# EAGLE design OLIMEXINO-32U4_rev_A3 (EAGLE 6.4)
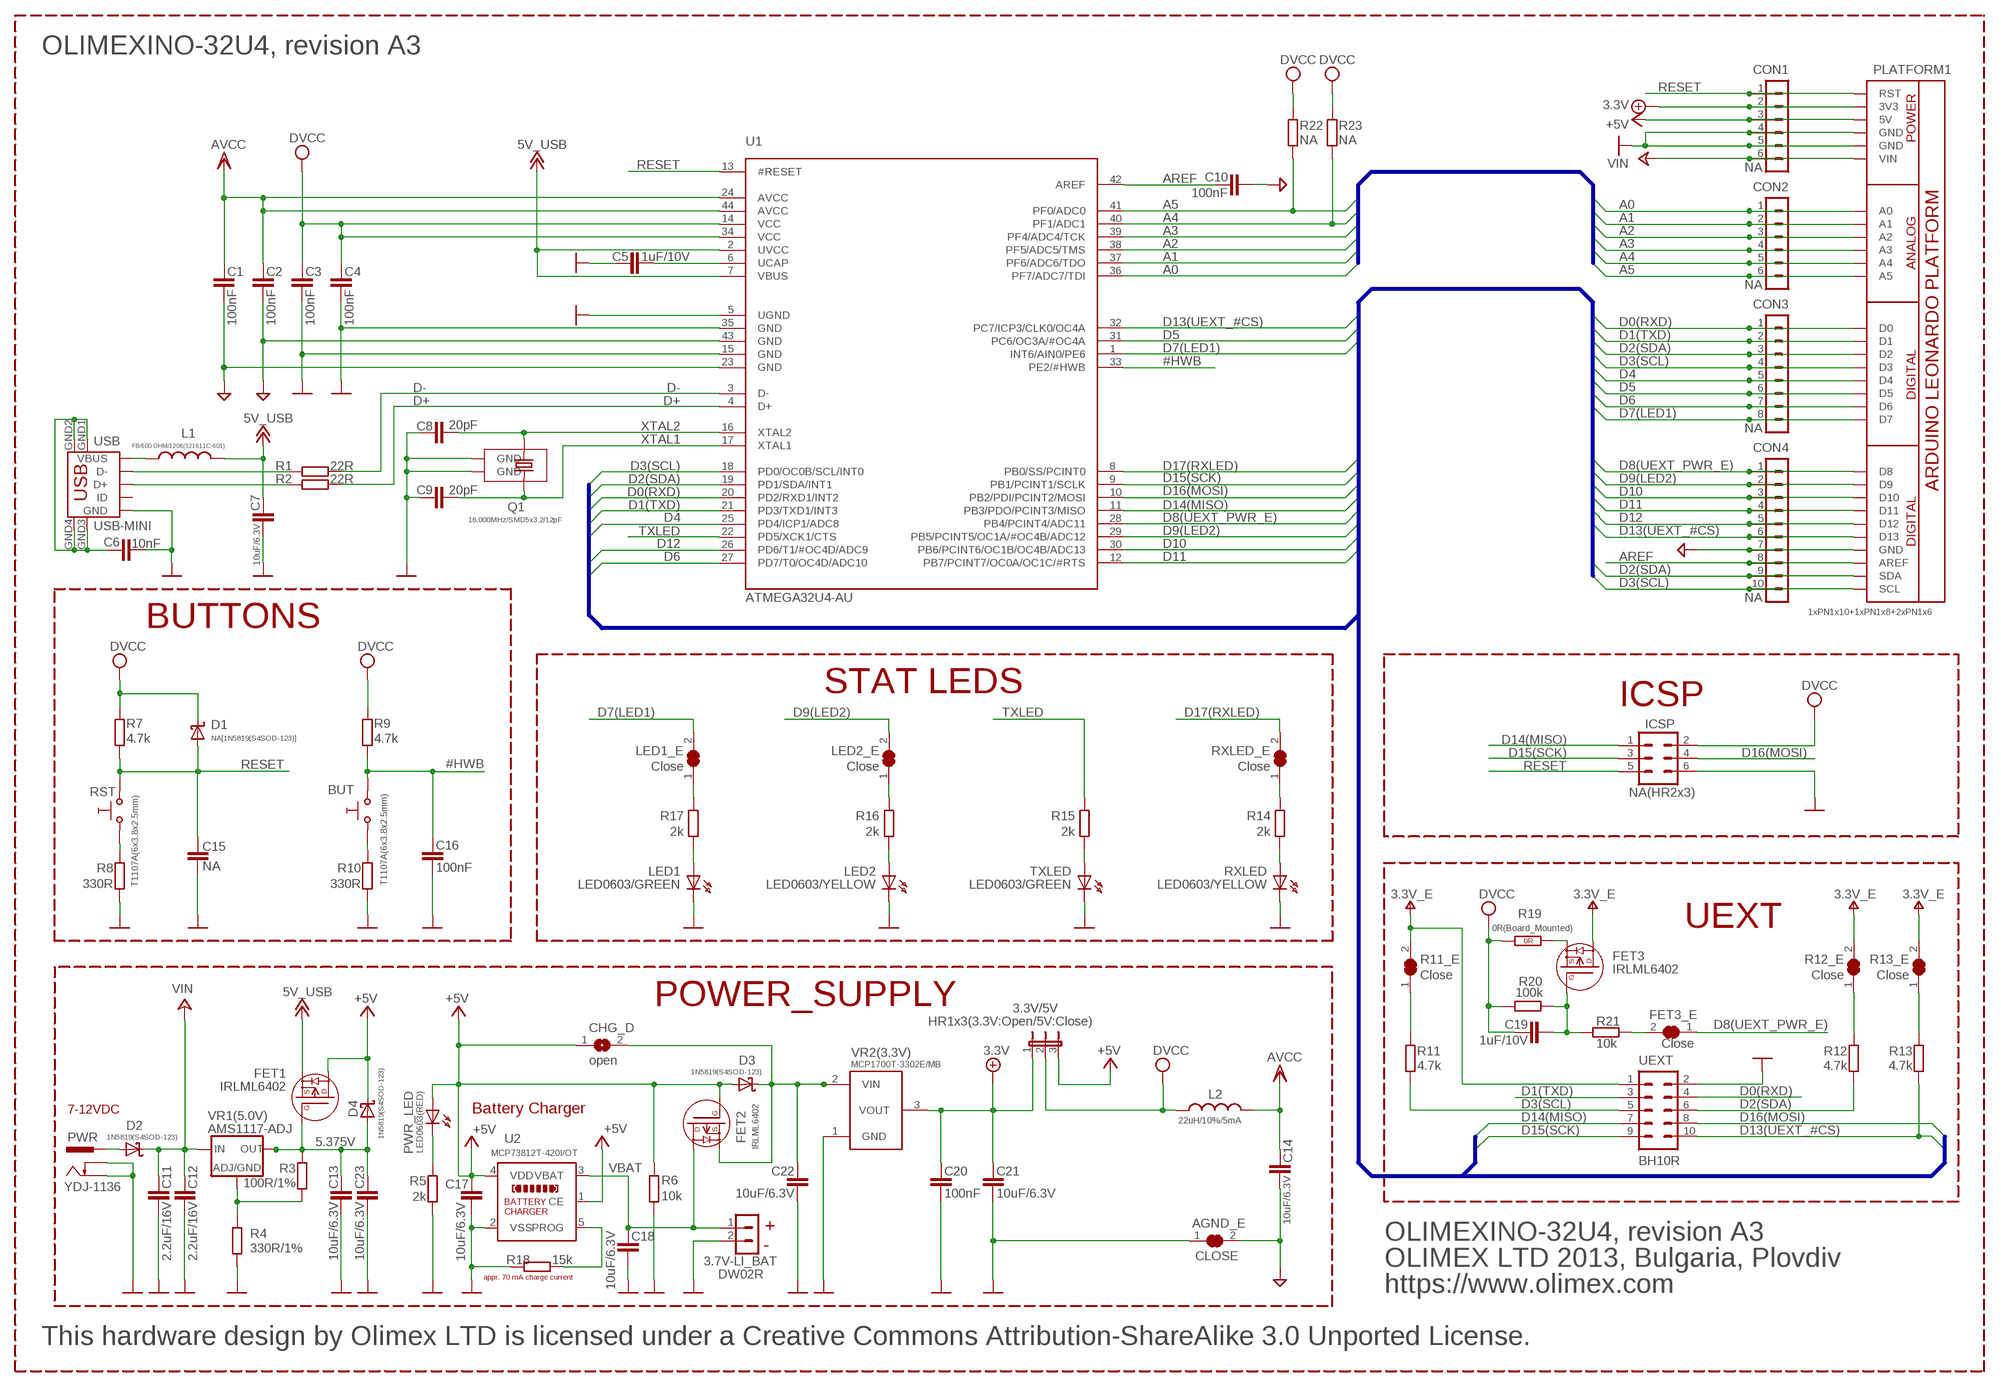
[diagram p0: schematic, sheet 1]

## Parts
3.3V/5V  HR1x3(3.3V:Open/5V:Close)  JP2EHR1X3  [HR1X3]
3.7V-LI_BAT  DW02R  CON2DW02R  [DW02R]
AGND_E  CLOSE  SJSJ_1_SMALLER_CLOSE  [SJ_1_SMALLER_CLOSE]
BUT  T1107A(6x3.8x2.5mm)  SW-TAKT6  [SW-TAKT_6X3.5_SMD]
C1  100nF  C-EUC0603_DWS  [C0603_DWS]
C2  100nF  C-EUC0603_DWS  [C0603_DWS]
C3  100nF  C-EUC0603_DWS  [C0603_DWS]
C4  100nF  C-EUC0603_DWS  [C0603_DWS]
C5  1uF/10V  C-EUC0603_DWS  [C0603_DWS]
C6  10nF  C-EUC0603_DWS  [C0603_DWS]
C7  10uF/6.3V  C-EUC0603_DWS  [C0603_DWS]
C8  20pF  C-EUC0603_DWS  [C0603_DWS]
C9  20pF  C-EUC0603_DWS  [C0603_DWS]
C10  100nF  C-EUC0603_DWS  [C0603_DWS]
C11  2.2uF/16V  C-EUC0805_5MIL_DWS  [C0805_5MIL_DWS]
C12  2.2uF/16V  C-EUC0805_5MIL_DWS  [C0805_5MIL_DWS]
C13  10uF/6.3V  C-EUC0603_DWS  [C0603_DWS]
C14  10uF/6.3V  C-EUC0603_DWS  [C0603_DWS]
C15  NA  C-EUC0603_DWS  [C0603_DWS]
C16  100nF  C-EUC0603_DWS  [C0603_DWS]
C17  10uF/6.3V  C-EUC0603_DWS  [C0603_DWS]
C18  10uF/6.3V  C-EUC0603_DWS  [C0603_DWS]
C19  1uF/10V  C-EUC0603_DWS  [C0603_DWS]
C20  100nF  C-EUC0603_DWS  [C0603_DWS]
C21  10uF/6.3V  C-EUC0603_DWS  [C0603_DWS]
C22  10uF/6.3V  C-EUC0603_DWS  [C0603_DWS]
C23  10uF/6.3V  C-EUC0603_DWS  [C0603_DWS]
CHG_D  open  SJSJ_SMALLER  [SJ_1_SMALLER]
CON1  NA  CON6HN1X6  [HN1X6]
CON2  NA  CON6HN1X6  [HN1X6]
CON3  NA  CON8HN1X8  [HN1X8]
CON4  NA  CON10HN1X10  [HN1X10]
D1  NA[1N5819(S4SOD-123)]  SCHOTKKY7.62SS-1N5819(S4SOD-123)  [SOD-123]
D2  1N5819(S4SOD-123)  SCHOTKKY7.62SS-1N5819(S4SOD-123)  [SOD-123]
D3  1N5819(S4SOD-123)  SCHOTKKY7.62SS-1N5819(S4SOD-123)  [SOD-123]
D4  1N5819(S4SOD-123)  SCHOTKKY7.62SS-1N5819(S4SOD-123)  [SOD-123]
FET1  IRLML6402  P-MOS+DIODIRLML6402  [SOT23]
FET2  IRLML6402  P-MOS+DIODIRLML6402  [SOT23]
FET3  IRLML6402  P-MOS+DIODIRLML6402  [SOT23]
FET3_E  Close  SJSJ_1_SMALLER_CLOSE  [SJ_1_SMALLER_CLOSE]
ICSP  NA(HR2x3)  ML6HN2X3R  [HN2X3R]
L1  FB/600 OHM/1206(321611C-601)  L-USL3216C  [L3216C]
L2  22uH/10%/5mA  L-USL3216C  [L3216C]
LED1  LED0603/GREEN  LED0603DWS  [LED-0603]
LED1_E  Close  SJSJ_1_SMALLER_CLOSE  [SJ_1_SMALLER_CLOSE]
LED2  LED0603/YELLOW  LED0603DWS  [LED-0603]
LED2_E  Close  SJSJ_1_SMALLER_CLOSE  [SJ_1_SMALLER_CLOSE]
PLATFORM1  1xPN1x10+1xPN1x8+2xPN1x6  ARDUINO_LEONARDO  [ARDUINO-LEONARDO-PLATFORM]
PWR  YDJ-1136  PWR-JAKPWR_JACK_UNI_MILLING  [PWR_JACK_UNI_MILLING]
PWR_LED  LED0603(RED)  LED0603DWS  [LED-0603]
Q1  16.000MHz/SMD5x3.2/12pF  SMALL_SMD_CRYSTAL  [CRYSTAL_SMD]
R1  22R  R-EU_R0603_5MIL_DWS  [R0603_5MIL_DWS]
R2  22R  R-EU_R0603_5MIL_DWS  [R0603_5MIL_DWS]
R3  100R/1%  R-EU_R0603_5MIL_DWS  [R0603_5MIL_DWS]
R4  330R/1%  R-EU_R0603_5MIL_DWS  [R0603_5MIL_DWS]
R5  2k  R-EU_R0603_5MIL_DWS  [R0603_5MIL_DWS]
R6  10k  R-EU_R0603_5MIL_DWS  [R0603_5MIL_DWS]
R7  4.7k  R-EU_R0603_5MIL_DWS  [R0603_5MIL_DWS]
R8  330R  R-EU_R0603_5MIL_DWS  [R0603_5MIL_DWS]
R9  4.7k  R-EU_R0603_5MIL_DWS  [R0603_5MIL_DWS]
R10  330R  R-EU_R0603_5MIL_DWS  [R0603_5MIL_DWS]
R11  4.7k  R-EU_R0603_5MIL_DWS  [R0603_5MIL_DWS]
R11_E  Close  SJSJ_1_SMALLER_CLOSE  [SJ_1_SMALLER_CLOSE]
R12  4.7k  R-EU_R0603_5MIL_DWS  [R0603_5MIL_DWS]
R12_E  Close  SJSJ_1_SMALLER_CLOSE  [SJ_1_SMALLER_CLOSE]
R13  4.7k  R-EU_R0603_5MIL_DWS  [R0603_5MIL_DWS]
R13_E  Close  SJSJ_1_SMALLER_CLOSE  [SJ_1_SMALLER_CLOSE]
R14  2k  R-EU_R0603_5MIL_DWS  [R0603_5MIL_DWS]
R15  2k  R-EU_R0603_5MIL_DWS  [R0603_5MIL_DWS]
R16  2k  R-EU_R0603_5MIL_DWS  [R0603_5MIL_DWS]
R17  2k  R-EU_R0603_5MIL_DWS  [R0603_5MIL_DWS]
R18  15k  R-EU_R0603_5MIL_DWS  [R0603_5MIL_DWS]
R19  0R(Board_Mounted)  R_0R0R(NA)  [0603_0R]
R20  100k  R-EU_R0603_5MIL_DWS  [R0603_5MIL_DWS]
R21  10k  R-EU_R0603_5MIL_DWS  [R0603_5MIL_DWS]
R22  NA  R-EU_R0603_5MIL_DWS  [R0603_5MIL_DWS]
R23  NA  R-EU_R0603_5MIL_DWS  [R0603_5MIL_DWS]
RST  T1107A(6x3.8x2.5mm)  SW-TAKT6  [SW-TAKT_6X3.5_SMD]
RXLED  LED0603/YELLOW  LED0603DWS  [LED-0603]
RXLED_E  Close  SJSJ_1_SMALLER_CLOSE  [SJ_1_SMALLER_CLOSE]
TXLED  LED0603/GREEN  LED0603DWS  [LED-0603]
U1  ATMEGA32U4-AU  ATMEGA32U4U  [TQFP44]
U2  MCP73812T-420I/OT  MCP7381XSOT-23-5  [SOT-23-5]
UEXT  BH10R  ML10R  [BH10R]
USB  USB-MINI  MINI_USB9  [USB_MINI_9PIN]
VR1(5.0V)  AMS1117-ADJ  LM1117  [SOT223]
VR2(3.3V)  MCP1700T-3302E/MB  MCP1700-REP1  [SOT89_REP_THERMALOFF]

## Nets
3.3V_REG_IN: C22.1 CHG_D.2 D3.C FET2.2(S) VR2(3.3V).2(VIN) VR2(3.3V).P$2(VIN1)
5.375V: C13.1 C23.1 D4.A FET1.1(G) R3.2 VR1(5.0V).2(OUT) VR1(5.0V).4(RAD)
#HWB: BUT.P$2 C16.1 R9.2 U1.33(PE2/#HWB)
+5V: 3.3V/5V.3 C17.1 CHG_D.1 CON1.3 D3.A D4.C FET1.3(D) FET2.1(G) PLATFORM1.5V PWR_LED.A R6.1 U2.1(CE) U2.4(VDD)
+5V/1: 3.3V/5V.1 C20.1 C21.1 CON1.2 PLATFORM1.3V3 VR2(3.3V).3(VOUT) ; supply symbol labelled 3.3V
+12V: C7.1 FET1.2(S) L1.2 U1.2(UVCC) U1.7(VBUS) ; supply symbol labelled 5V_USB
+24V: C11.1 C12.1 CON1.6 D2.C PLATFORM1.VIN VR1(5.0V).3(IN) ; supply symbol labelled VIN
A0: CON2.1 PLATFORM1.A0 U1.36(PF7/ADC7/TDI)
A1: CON2.2 PLATFORM1.A1 U1.37(PF6/ADC6/TDO)
A2: CON2.3 PLATFORM1.A2 U1.38(PF5/ADC5/TMS)
A3: CON2.4 PLATFORM1.A3 U1.39(PF4/ADC4/TCK)
A4: CON2.5 PLATFORM1.A4 R23.1 U1.40(PF1/ADC1)
A5: CON2.6 PLATFORM1.A5 R22.1 U1.41(PF0/ADC0)
AGND: AGND_E.2 C1.2 C2.2 C10.2 C14.2 CON4.7 PLATFORM1.GND@2(GND) U1.23(GND) U1.43(GND)
AREF: C10.1 CON4.8 PLATFORM1.AREF U1.42(AREF)
D0(RXD): CON3.1 PLATFORM1.D0 U1.20(PD2/RXD1/INT2) UEXT.4
D1(TXD): CON3.2 PLATFORM1.D1 U1.21(PD3/TXD1/INT3) UEXT.3
D2(SDA): CON3.3 CON4.9 PLATFORM1.D2 PLATFORM1.SDA R12.1 U1.19(PD1/SDA/INT1) UEXT.6
D3(SCL): CON3.4 CON4.10 PLATFORM1.D3 PLATFORM1.SCL R11.1 U1.18(PD0/OC0B/SCL/INT0) UEXT.5
D4: CON3.5 PLATFORM1.D4 U1.25(PD4/ICP1/ADC8)
D5: CON3.6 PLATFORM1.D5 U1.31(PC6/OC3A/#OC4A)
D6: CON3.7 PLATFORM1.D6 U1.27(PD7/T0/OC4D/ADC10)
D7(LED1): CON3.8 LED1_E.2 PLATFORM1.D7 U1.1(INT6/AIN0/PE6)
D8(UEXT_PWR_E): CON4.1 FET3_E.1 PLATFORM1.D8 U1.28(PB4/PCINT4/ADC11)
D9(LED2): CON4.2 LED2_E.2 PLATFORM1.D9 U1.29(PB5/PCINT5/OC1A/#OC4B/ADC12)
D10: CON4.3 PLATFORM1.D10 U1.30(PB6/PCINT6/OC1B/OC4B/ADC13)
D11: CON4.4 PLATFORM1.D11 U1.12(PB7/PCINT7/OC0A/OC1C/#RTS)
D12: CON4.5 PLATFORM1.D12 U1.26(PD6/T1/#OC4D/ADC9)
D13(UEXT_#CS): CON4.6 PLATFORM1.D13 R13.1 U1.32(PC7/ICP3/CLK0/OC4A) UEXT.10
D14(MISO): ICSP.1 U1.11(PB3/PDO/PCINT3/MISO) UEXT.7
D15(SCK): ICSP.3 U1.9(PB1/PCINT1/SCLK) UEXT.9
D16(MOSI): ICSP.4 U1.10(PB2/PDI/PCINT2/MOSI) UEXT.8
D17(RXLED): RXLED_E.2 U1.8(PB0/SS/PCINT0)
D+: R2.2 U1.4(D+)
D-: R1.2 U1.3(D-)
GND [pwr]: 3.7V-LI_BAT.2 AGND_E.1 C3.2 C4.2 C5.1 C6.2 C7.2 C8.1 C9.1 C11.2 C12.2 C13.2 C15.2 C16.2 C17.2 C18.2 C20.2 C21.2 C22.2 C23.2 CON1.4 CON1.5 ICSP.6 LED1.C LED2.C PLATFORM1.GND PLATFORM1.GND@1(GND) PWR.- PWR.-- Q1.NC_1(GND) Q1.NC_2(GND) R4.1 R5.2 R6.2 R8.1 R10.1 R18.1 RXLED.C TXLED.C U1.5(UGND) U1.15(GND) U1.35(GND) U2.2(VSS) UEXT.2 USB.GND VR2(3.3V).1(GND)
N$1: R1.1 USB.D-
N$2: R14.2 RXLED_E.1
N$3: R2.1 USB.D+
N$4: R11.2 R11_E.1
N$5: R15.1 TXLED.A
N$6: FET3_E.2 R21.2
N$8: R13.2 R13_E.1
N$9: LED1.A R17.1
N$11 [pwr]: R8.2 RST.P$2
N$12: BUT.P$1 R10.2
N$13: R12.2 R12_E.1
N$15: LED1_E.1 R17.2
N$16: D2.A PWR.+
N$17: LED2.A R16.1
N$18: LED2_E.1 R16.2
N$19: C19.2 FET3.1(G) R20.2 R21.1
N$20: FET3.2(S) R19.2(1.2)
N$21: PWR_LED.C R5.1
N$22: R18.2 U2.5(PROG)
N$23: R14.1 RXLED.A
N$118: C6.1 USB.GND1 USB.GND2 USB.GND3 USB.GND4
RESET: C15.1 CON1.1 D1.A ICSP.5 PLATFORM1.RST R7.2 RST.P$1 U1.13(#RESET)
TXLED: R15.2 U1.22(PD5/XCK1/CTS)
UCAP: C5.2 U1.6(UCAP)
V+: FET3.3(D) R11_E.2 R12_E.2 R13_E.2 UEXT.1 ; supply symbol labelled 3.3V_E
VBAT: 3.7V-LI_BAT.1 C18.1 FET2.3(D) U2.3(VBAT)
VBUS: L1.1 USB.VBUS
VCC: 3.3V/5V.2 C3.1 C4.1 C19.1 D1.C ICSP.2 L2.1 R7.1 R9.1 R19.1(1.1) R20.1 R22.2 R23.2 U1.14(VCC) U1.34(VCC) ; supply symbol labelled DVCC
VDD: C1.1 C2.1 C14.1 L2.2 U1.24(AVCC) U1.44(AVCC) ; supply symbol labelled AVCC
VR1_ADJ: R3.1 R4.2 VR1(5.0V).1(ADJ/GND)
XTAL1: C9.2 Q1.1 U1.17(XTAL1)
XTAL2: C8.2 Q1.2 U1.16(XTAL2)
Unconnected: USB.ID

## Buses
A[0..5]
D0(RXD),D1(TXD),D2(SDA),D3(SCL),D[4..6],D7(LED1),D8(UEXT_PWR_E),D9(LED2),D[10..12],D13(UEXT_#CS),D14(RXLED),D15(SCK),D16(MOSI),D17(MISO)

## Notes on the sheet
- OLIMEXINO-32U4, revision A3
- BUTTONS
- STAT LEDS
- ICSP
- UEXT
- POWER_SUPPLY
- 7-12VDC | Battery Charger
- +
- - | OLIMEXINO-32U4, revision A3
- OLIMEX LTD 2013, Bulgaria, Plovdiv
- appr. 70 mA charge current
- https://www.olimex.com
- This hardware design by Olimex LTD is licensed under a Creative Commons Attribution-ShareAlike 3.0 Unported License.

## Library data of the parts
3.3V/5V = jumper:JP2E: JUMPER
3.7V-LI_BAT = Penko:CON2
AGND_E CHG_D FET3_E LED1_E LED2_E R11_E R12_E R13_E RXLED_E = jumper:SJ: SMD solder JUMPER
BUT RST = gogo:SW-TAKT
C1-C23 = rcl:C-EU: CAPACITOR, European symbol
CON1 CON2 = Penko:CON6: CONNECTORS - 6 PINS
CON3 = Penko:CON8
CON4 = Penko:CON10
D1-D4 = gogo:SCHOTKKY7.62SS
FET1-FET3 = Penko:P-MOS+DIOD
ICSP = con-harting-ml:ML6: HARTING
L1 L2 = rcl:L-US: INDUCTOR, American symbol
LED1 LED2 PWR_LED RXLED TXLED = DOUBLE-SIDE:LED
PLATFORM1 = OLIMEX_CASES:ARDUINO_LEONARDO
PWR = gogo:PWR-JAK
Q1 = OLIMEX_DISCRET:SMALL_SMD_CRYSTAL
R1-R18 R20-R23 = rcl:R-EU_: RESISTOR, European symbol
R19 = OLIMEX_DISCRET:R_0R
U1 = OLIMEX_IC:ATMEGA32U4: 8-bit Microcontroller with 16/32K Bytes of ISP Flash and USB Controller
U2 = OLIMEX_DISCRET:MCP7381X
UEXT = con-harting-ml:ML10: HARTING
USB = OLIMEX_CONNECTORS:MINI_USB9
VR1(5.0V) = arm:LM1117
VR2(3.3V) = OLIMEX_DISCRET:MCP1700-REP

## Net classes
1 pwr: width 0.25 mm

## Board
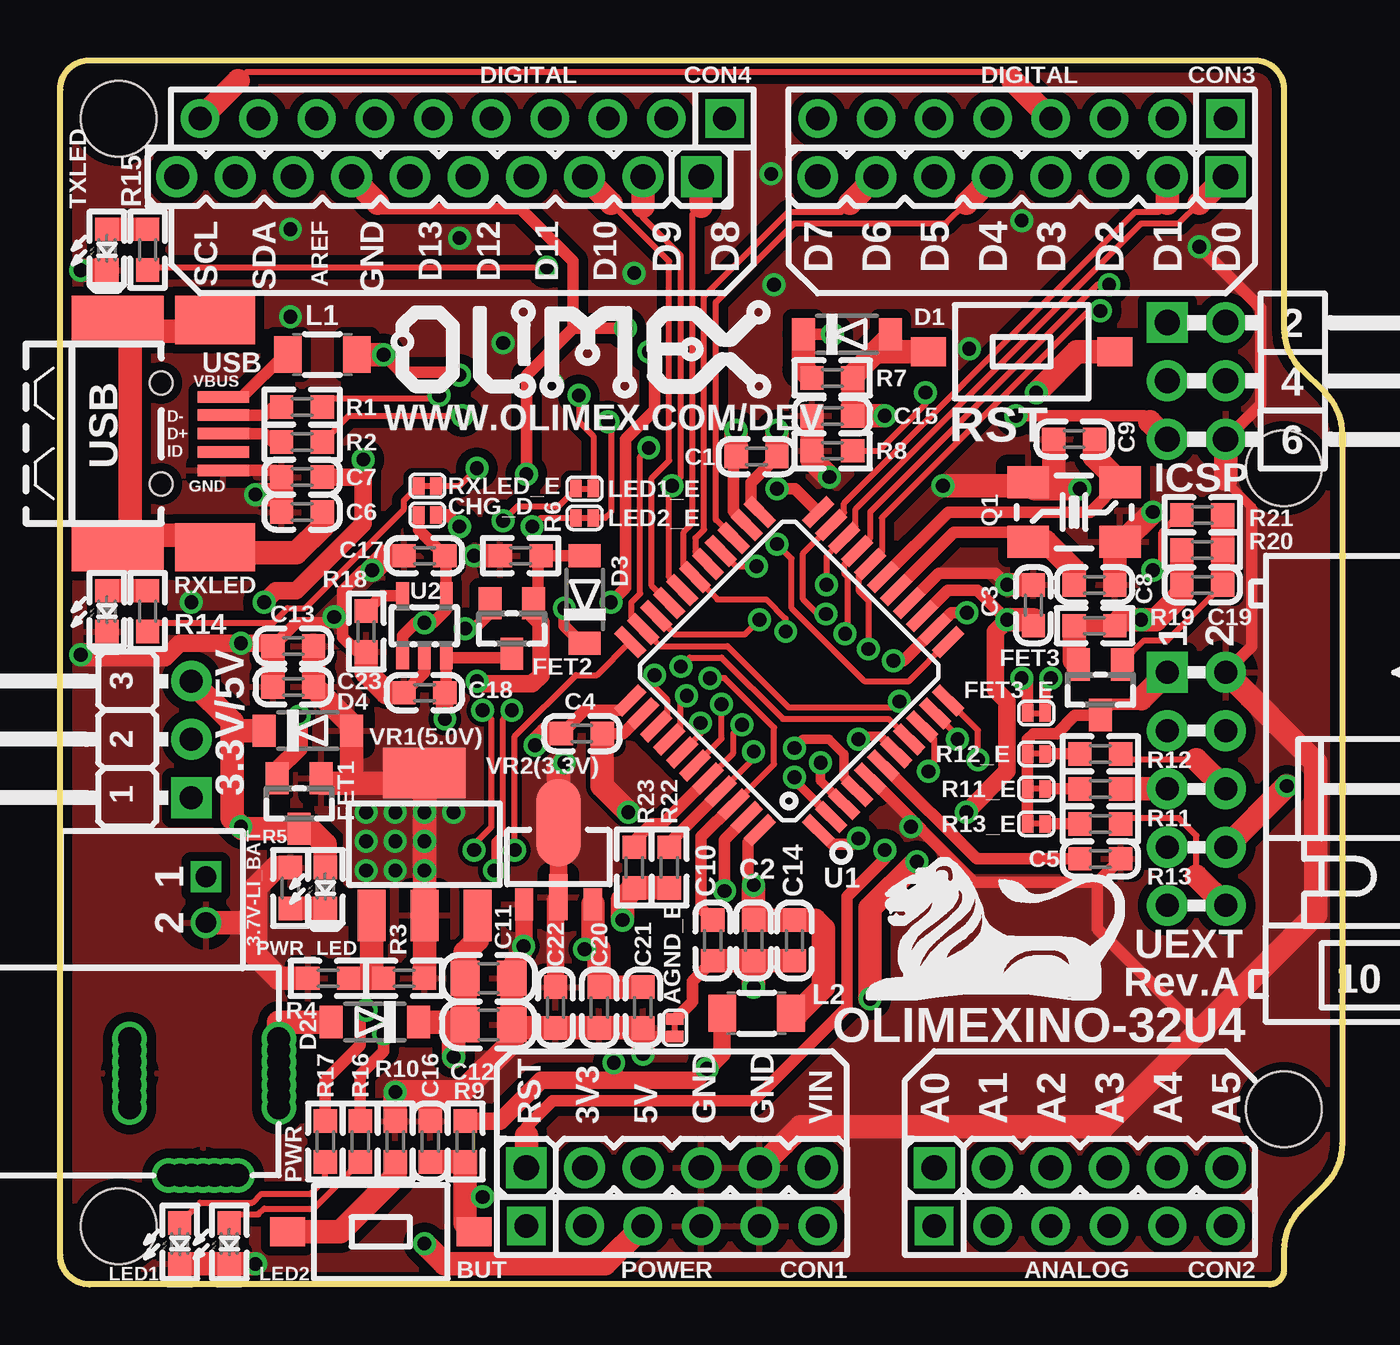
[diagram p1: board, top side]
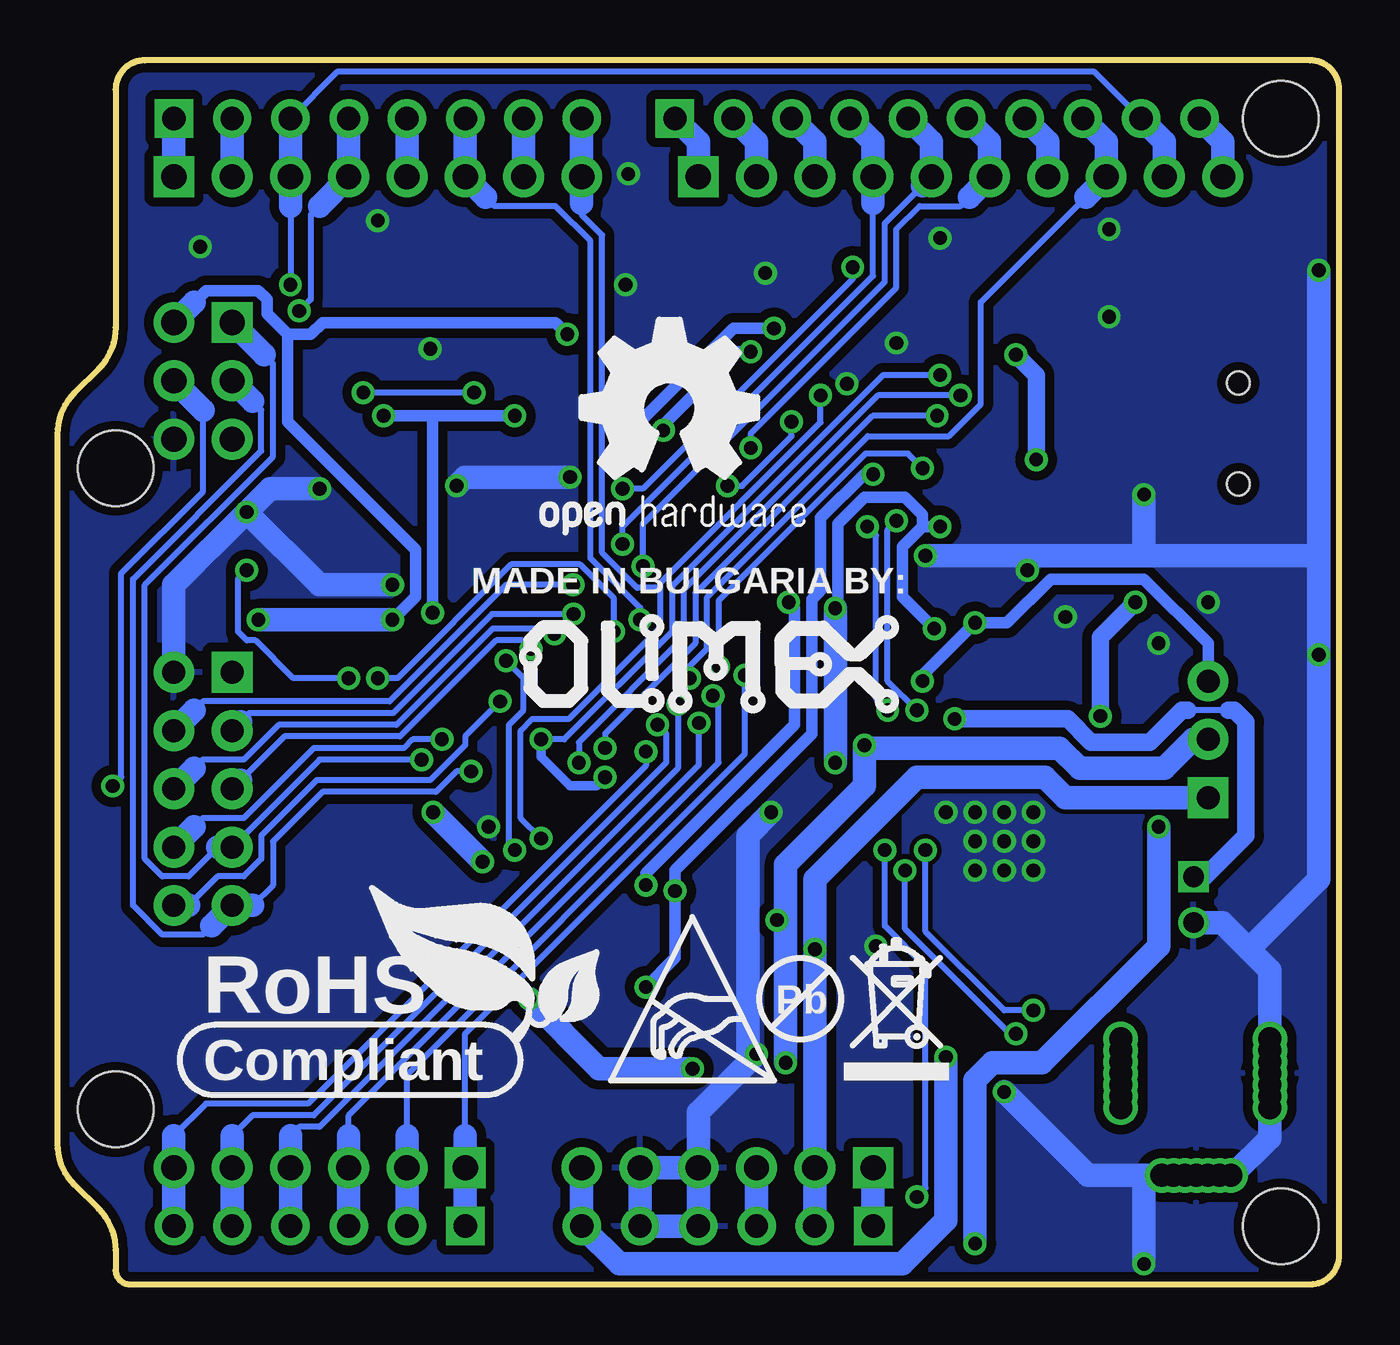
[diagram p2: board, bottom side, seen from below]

Size 55.88 x 53.34 mm. Coordinates in mm from the lower left corner, seen from the top.
Copper layers (1+16): Top 0.035mm / dielectric 1.5mm / Bottom 0.035mm
Design rules "default": minimum track width 10mil, minimum drill 0.6mm, track to track 0.2mm, track to pad 0.2mm, pad to pad 0.2mm, via to via 0.2mm, smd to smd 1mil, copper to edge 10mil, drill to drill 8mil, minimum pad ring 8mil, minimum via ring 0.2mm, stop-mask expansion 4mil, vias tented up to drill 25mil, thermal gap 20mil

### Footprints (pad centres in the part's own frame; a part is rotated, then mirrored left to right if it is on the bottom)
HR1X3 = drill 1 pad 1.778 square: 1 -2.54,0 | drill 1 pad 1.778: 2 0,0; 3 2.54,0
DW02R = drill 0.9 square: 1 -1,0 | drill 0.9: 2 1,0
SJ_1_SMALLER_CLOSE = smd 0.508 x 0.762: 1 -0.381,0; 2 0.381,0
SW-TAKT_6X3.5_SMD = smd 1.27 x 1.524: P$1 0,4.064; P$2 0,-4.064
C0603_DWS = smd 1.016 x 1.016: 1 -0.889,0; 2 0.889,0
C0805_5MIL_DWS = smd 1.27 x 1.524: 1 -1.016,0; 2 1.016,0
SJ_1_SMALLER = smd 0.508 x 0.762: 1 -0.381,0; 2 0.381,0
HN1X6 = drill 1.1 pad 1.778 square: 1 -6.35,0 | drill 1.1 pad 1.778: 2 -3.81,0; 3 -1.27,0; 4 1.27,0; 5 3.81,0; 6 6.35,0
HN1X8 = drill 1.1 pad 1.778 square: 1 -8.89,0 | drill 1.1 pad 1.778: 2 -6.35,0; 3 -3.81,0; 4 -1.27,0; 5 1.27,0; 6 3.81,0; 7 6.35,0; 8 8.89,0
HN1X10 = drill 1.1 pad 1.778 square: 1 -11.43,0 | drill 1.1 pad 1.778: 2 -8.89,0; 3 -6.35,0; 4 -3.81,0; 5 -1.27,0; 6 1.27,0; 7 3.81,0; 8 6.35,0; 9 8.89,0; 10 11.43,0
SOD-123 = smd 1 x 1.4: A 1.9,0; C -1.9,0
SOT23 = smd 1 x 1.4: 1 -0.95,-1.1; 2 0.95,-1.1; 3 0,1.1
HN2X3R = drill 1.1 pad 1.778 square: 1 -2.54,-1.27 | drill 1.1 pad 1.778: 2 -2.54,1.27; 3 0,-1.27; 4 0,1.27; 5 2.54,-1.27; 6 2.54,1.27
L3216C = smd 1.2 x 1.6: 1 -1.5,0; 2 1.5,0
LED-0603 = smd 1.016 x 1.016: A 0.889,0; C -0.889,0
ARDUINO-LEONARDO-PLATFORM = drill 1.016 pad 1.676: 3V3 22.86,2.54; 5V 25.4,2.54; A1 40.64,2.54; A2 43.18,2.54; A3 45.72,2.54; A4 48.26,2.54; A5 50.8,2.54; AREF 11.176,50.8; D1 48.26,50.8; D2 45.72,50.8; D3 43.18,50.8; D4 40.64,50.8; D5 38.1,50.8; D6 35.56,50.8; D7 33.02,50.8; D9 26.416,50.8; D10 23.876,50.8; D11 21.336,50.8; D12 18.796,50.8; D13 16.256,50.8; GND 27.94,2.54; GND@1 30.48,2.54; GND@2 13.716,50.8; SCL 6.096,50.8; SDA 8.636,50.8; VIN 33.02,2.54 | drill 1.016 pad 1.676 square: A0 38.1,2.54; D0 50.8,50.8; D8 28.956,50.8; RST 20.32,2.54 | hole 3.3: 53.34,35.56; 53.34,7.62; 2.54,50.8; 2.54,2.54
PWR_JACK_UNI_MILLING = drill 1: + 0,4.75; +1 0,5.25; +2 0,5.75; +3 0,6.25; +4 0,4.25; +5 0,3.75; +6 0,3.25; - -6.5,4.75; -1 -6.5,5.25; -2 -6.5,5.75; -3 -6.5,4.25; -4 -6.5,3.75; -5 -6.5,6.25; -6 -6.5,3.25; -- -3.3,0.3; --1 -3.8,0.3; --2 -4.3,0.3; --3 -4.8,0.3; --4 -2.8,0.3; --5 -2.3,0.3; --6 -1.8,0.3
CRYSTAL_SMD = smd 1.8 x 1.4: 1 -2,-1.3; 2 2,1.3; NC_1 2,-1.3; NC_2 -2,1.3
R0603_5MIL_DWS = smd 1.016 x 1.016: 1 -0.889,0; 2 0.889,0
0603_0R = smd 1.016 x 1.016: 1 -0.889,0; 2 0.889,0
TQFP44 = smd 1.5 x 0.5: 1 -5.78,3.95; 2 -5.78,3.15; 3 -5.78,2.35; 4 -5.78,1.55; 5 -5.78,0.75; 6 -5.78,-0.05; 7 -5.78,-0.85; 8 -5.78,-1.65; 9 -5.78,-2.45; 10 -5.78,-3.25; 11 -5.78,-4.05; 23 5.82,-4.05; 24 5.82,-3.25; 25 5.82,-2.45; 26 5.82,-1.65; 27 5.82,-0.85; 28 5.82,-0.05; 29 5.82,0.75; 30 5.82,1.55; 31 5.82,2.35; 32 5.82,3.15; 33 5.82,3.95 | smd 0.5 x 1.5: 12 -3.98,-5.85; 13 -3.18,-5.85; 14 -2.38,-5.85; 15 -1.58,-5.85; 16 -0.78,-5.85; 17 0.02,-5.85; 18 0.82,-5.85; 19 1.62,-5.85; 20 2.42,-5.85; 21 3.22,-5.85; 22 4.02,-5.85; 34 4.02,5.75; 35 3.22,5.75; 36 2.42,5.75; 37 1.62,5.75; 38 0.82,5.75; 39 0.02,5.75; 40 -0.78,5.75; 41 -1.58,5.75; 42 -2.38,5.75; 43 -3.18,5.75; 44 -3.98,5.75
SOT-23-5 = smd 0.55 x 1.2: 1 -0.95,-1.3; 2 0,-1.3; 3 0.95,-1.3; 4 0.95,1.3; 5 -0.95,1.3
BH10R = drill 1 pad 1.778 square: 1 -5.08,-1.27 | drill 1 pad 1.778: 2 -5.08,1.27; 3 -2.54,-1.27; 4 -2.54,1.27; 5 0,-1.27; 6 0,1.27; 7 2.54,-1.27; 8 2.54,1.27; 9 5.08,-1.27; 10 5.08,1.27
USB_MINI_9PIN = smd 2.25 x 0.5: D+ 2.706,0; D- 2.706,0.8; GND 2.706,-1.6; ID 2.706,-0.8; VBUS 2.706,1.6 | smd 4 x 2.1: GND1 -1.9,4.95; GND3 -1.9,-4.95 | smd 3.5 x 2.1: GND2 2.35,4.95; GND4 2.35,-4.95 | hole 1: 0,2.2; 0,-2.2
SOT223 = smd 1.219 x 2.235: 1 -2.311,-3.099; 2 0,-3.099; 3 2.311,-3.099 | smd 3.6 x 2.2: 4 0,3.099
SOT89_REP_THERMALOFF = smd 0.8 x 1.4: 1 -1.499,-1.981; 3 1.499,-1.981 | smd 0.8 x 2: 2 0,-1.681 | smd 1.93 x 3.81: P$2 0,1.57

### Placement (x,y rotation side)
3.3V/5V  5.71,23.75 90 top
3.7V-LI_BAT  6.35,16.76 270 top
AGND_E  26.8,11.18 90 top
BUT  13.97,2.29 90 top
C1  30.35,36.07 0 top
C2  30.23,14.99 270 top
C3  42.42,29.59 90 top
C4  22.73,24 0 top
C5  45.34,18.54 180 top
C6  10.54,33.66 180 top
C7  10.54,35.18 180 top
C8  45.09,30.48 180 top
C9  44.2,36.83 0 top
C10  28.45,14.99 270 top
C11  18.67,13.34 0 top
C12  18.67,11.3 0 top
C13  10.16,27.81 180 top
C14  32,14.99 270 top
C15  33.66,37.85 180 top
C16  16.13,6.22 90 top
C17  15.88,31.75 180 top
C18  15.88,25.78 180 top
C19  49.78,30.48 0 top
C20  23.5,12.06 270 top
C21  25.4,12.06 270 top
C22  21.59,12.06 270 top
C23  10.16,26.04 180 top
CHG_D  16,33.53 0 top
CON1  26.67,5.08 0 top
CON2  44.45,5.08 0 top
CON3  41.91,48.26 180 top
CON4  16.51,48.26 180 top
D1  34.29,41.4 0 top
D2  13.72,11.43 180 top
D3  22.86,29.84 90 top
D4  10.79,24.13 0 top
FET1  10.41,20.95 180 top
FET2  19.68,28.57 180 top
FET3  45.34,25.91 180 top
FET3_E  42.55,24.89 0 top
ICSP  49.53,39.37 270 top
L1  11.43,40.51 0 top
L2  30.35,11.81 0 top
LED1  5.21,1.78 90 top
LED1_E  22.86,34.67 0 top
LED2  7.37,1.78 90 top
LED2_E  22.86,33.4 0 top
PLATFORM1  0,0 0 top
PWR  9.53,4.45 0 top
PWR_LED  11.56,17.27 90 top
Q1  44.2,33.66 180 top
R1  10.54,38.23 0 top
R2  10.54,36.7 0 top
R3  14.99,13.34 0 top
R4  11.68,13.34 0 top
R5  10.03,17.27 90 top
R6  20.07,31.75 180 top
R7  33.66,39.5 0 top
R8  33.66,36.32 0 top
R9  17.65,6.22 270 top
R10  14.61,6.22 270 top
R11  45.34,21.59 180 top
R11_E  42.55,21.59 180 top
R12  45.34,23.11 180 top
R12_E  42.55,23.11 180 top
R13  45.34,20.07 180 top
R13_E  42.55,20.07 180 top
R14  3.81,29.34 270 top
R15  3.81,45.09 270 top
R16  13.08,6.22 90 top
R17  11.56,6.22 90 top
R18  13.34,28.45 90 top
R19  45.09,28.7 180 top
R20  49.78,32 0 top
R21  49.78,33.53 180 top
R22  26.54,18.16 270 top
R23  25.02,18.16 270 top
RST  41.91,40.64 90 top
RXLED  2.03,29.34 90 top
RXLED_E  16,34.8 0 top
TXLED  2.03,45.09 90 top
U1  31.75,26.67 135 top
U2  15.88,28.7 0 top
U$1  [RECYCLE_BIN1/8]  21.59,8.89 0 bottom
U$2  [PB_SMALL]  23.5,12.45 0 bottom
U$3  [LOGO-OPENHARDWARE_8X8]  29.21,38.1 0 bottom
U$8  [ROHS]  49.53,8.89 0 bottom
U$9  [OLIMEX1_V]  32.13,38.48 0 top
U$10  [LION_12X7MM]  40.39,13.97 0 top
U$11  [ESD_SYMBOL]  31.75,8.89 0 bottom
U$12  [OLIMEX1_V]  18.03,24.77 0 bottom
UEXT  49.53,21.59 270 top
USB  4.4,37.07 0 top
VR1(5.0V)  15.88,19.18 0 top
VR2(3.3V)  21.72,18.54 0 top

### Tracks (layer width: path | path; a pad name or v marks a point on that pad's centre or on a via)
3.3V_REG_IN  (via drill 0.6)
  Top 0.508: v17.4,33.02 16.89,33.53 CHG_D.2 | FET2.2 18.73,29.28 18.03,28.57 v17.65,28.57 | D3.C 22.73,27.95 21.97,28.7 v21.97,29.46
  Top 0.762: VR2(3.3V).P$2 VR2(3.3V).2 21.59,16.73 C22.1
  Top 1.016: VR2(3.3V).P$2 21.72,22.48 v21.97,22.73
  Bottom 0.508: 18.16,33.02 19.05,32.13 19.05,29.97 v17.65,28.57 | 18.16,33.02 v17.4,33.02 | v21.97,29.46 21.84,29.59 21.84,33.15 20.7,34.29 18.92,34.29 18.16,33.53 18.16,33.02
  Bottom 1.016: v21.97,22.73 v21.97,29.46
  pour Top: 19.68,17.53 20.45,17.53 20.7,17.27 20.7,12.19 20.83,12.06 22.35,12.06 22.61,12.32 22.61,17.4 22.86,17.65 24.26,17.65 24.38,17.78 24.38,22.48 22.99,23.88 20.95,23.88 19.56,22.48 19.56,17.53
5.375V  (via drill 0.6)
  Top 1.016: C13.1 C23.1 12.7,24.38 D4.A 12.7,21.84 | 15.88,21.84 v15.88,20.57 v15.88,19.3 v15.88,18.03 VR1(5.0V).2 R3.2 | 15.88,21.84 VR1(5.0V).4 | 15.88,21.84 12.7,21.84 | FET1.1 11.36,21.84 12.7,21.84
  other vias: 17.14,20.57 14.61,20.57 14.61,19.3 13.34,19.3 13.34,20.57 14.61,18.03 13.34,18.03
  pour Top: 10.16,28.45 10.16,25.27 10.92,24.64 10.92,23.11 10.16,22.35 10.16,20.57 10.41,20.32 11.81,20.32 12.45,19.68 12.45,17.53 12.57,17.4 13.08,17.4 13.34,17.14 13.34,13.08 13.84,12.57 16.64,12.57 17.65,13.59 17.65,17.14 17.91,17.4 18.67,17.4 19.05,17.78 19.05,24.51 17.91,25.65 13.97,25.65 12.95,26.67 12.95,27.94 12.06,28.83 10.54,28.83
  pour Bottom: 14.99,12.06 18.92,16 18.92,22.73 13.21,22.73 12.06,21.59 9.02,21.59 7.87,20.45 7.87,14.61 10.41,12.06
#HWB  (via drill 0.6)
  Top 0.254: 17.65,3.81 v18.41,3.81 | U1.33 23.39,26.54 22.48,26.54 19.81,23.88 v19.81,18.92
  Top 1.016: C16.1 R9.2 17.65,3.81 17.65,2.67 BUT.P$2
  Bottom 0.254: v18.41,3.81 18.03,4.19 18.03,13.84 19.81,15.62 v19.81,18.92
+5V  (via drill 0.6)
  Top 0.508: U2.1 14.93,28.26 15.49,28.83 v15.88,28.83 16.26,28.83 16.82,29.4 U2.4 16.82,31.69 C17.1 15.62,32.89 CHG_D.1 | FET2.1 20.83,29.68 20.83,31.5 21.08,31.75 | D3.A 21.08,31.75 | 21.08,31.75 R6.1
  Top 0.762: 7.49,24.51 7.49,24.26 7.49,24.13 | FET2.1 20.64,29.15 20.95,28.83 20.95,26.54 20.57,26.16 18.29,26.16 v18.16,26.29
  Top 1.016: 7.49,24.13 D4.C | 7.49,24.51 3.3V/5V.3 | PLATFORM1.5V 23.75,0.89 16.76,0.89 v15.88,1.78 | 7.49,24.26 7.49,20.32 v7.87,19.94 7.96,19.86 FET1.3 10.88,19.86 11.56,19.18 PWR_LED.A
  Bottom 0.508: 3.3V/5V.3 5.71,27.94 8.51,30.73 12.57,30.73 14.48,28.83 v15.88,28.83 18.16,26.54 v18.16,26.29
  Bottom 1.016: PLATFORM1.5V CON1.3 | v15.88,1.78 15.88,8.89 15.11,9.65 12.95,9.65 7.87,14.73 v7.87,19.94
+5V/1  (via drill 0.6)
  Top 1.016: C21.1 C20.1 23.5,14.61 23.22,14.61 | 23.22,14.61 VR2(3.3V).3 | v22.86,14.61 23.22,14.61
  Bottom 1.016: PLATFORM1.3V3 CON1.2 v22.86,14.61 22.86,17.65 18.41,22.1 12.83,22.1 11.94,21.21 3.3V/5V.1
+12V  (via drill 0.6)
  Top 0.406: U1.7 35.75,23.88 34.92,23.88 v34.8,23.75 | U1.2 32,21.96 v32,22.1
  Top 0.508: v14.1,40.51 14.86,39.75 17.27,39.75 v17.4,39.62
  Top 0.762: 13.21,35.18 13.21,33.15 10.29,30.23 9.4,30.23 v8.89,29.72 | 13.21,35.18 v13.21,35.94 | 13.21,35.18 C7.1 | FET1.2 9.46,22.42 10.41,23.37 v10.41,24.77
  Top 1.016: v14.1,40.51 L1.2
  Bottom 0.254: v34.8,23.75 33.78,23.75 29.08,28.45 29.08,30.43 19.89,39.62 v17.4,39.62
  Bottom 0.406: v32,22.1 32.38,21.72 33.53,21.72 34.8,22.99 v34.8,23.75
  Bottom 0.762: v14.1,40.51 13.21,39.62 v13.21,35.94 | v10.41,24.77 10.41,28.19 v8.89,29.72
+24V  (via drill 0.6)
  Top 1.016: 17.65,11.43 C11.1 17.65,14.48 18.19,15.01 VR1(5.0V).3 | 17.14,11.43 17.65,11.43 | 17.65,11.43 C12.1 | v17.14,9.91 17.14,11.43 | 17.14,11.43 D2.C
  Bottom 1.016: CON1.6 PLATFORM1.VIN 31.37,0.89 19.05,0.89 17.14,2.79 v17.14,9.91
A0  (via drill 0.6)
  Top 0.254: U1.36 26.44,24.78 26.44,25.5 25.91,26.04 v25.91,26.54
  Bottom 0.254: v25.91,26.54 25.91,23.11 38.1,10.92 38.1,6.48
  Bottom 1.016: PLATFORM1.A0 CON2.1 38.1,6.48
A1  (via drill 0.6)
  Top 0.254: U1.37 27.03,24.24 27.03,25.38 v27.3,25.65
  Bottom 0.254: v27.3,25.65 27.05,25.4 27.05,22.73 40.64,9.14 40.64,6.48
  Bottom 1.016: PLATFORM1.A1 CON2.2 40.64,6.48
A2  (via drill 0.6)
  Top 0.254: U1.38 27.91,23.99 v27.91,24.46
  Bottom 0.254: v27.91,24.46 27.91,22.63 43.18,7.37 43.18,6.48
  Bottom 1.016: PLATFORM1.A2 CON2.3 43.18,6.48
A3  (via drill 0.6)
  Top 0.254: U1.39 28.83,23.78 v28.83,25.27
  Bottom 0.254: v28.83,25.27 28.83,22.48 44.45,6.86 45.34,6.86 45.72,6.48
  Bottom 1.016: PLATFORM1.A3 CON2.4 45.72,6.48
A4  (via drill 0.6)
  Top 0.254: U1.40 29.34,23.15 29.34,24 v29.72,24.38
  Top 0.508: U1.40 26.25,20.07 25.78,20.07 25.02,19.3 R23.1
  Bottom 0.254: v29.72,24.38 29.34,24 29.34,22.73 44.7,7.37 47.37,7.37 48.26,6.48
  Bottom 1.016: PLATFORM1.A4 CON2.5 48.26,6.48
A5  (via drill 0.6)
  Top 0.254: U1.41 30.23,22.91 v30.23,23.22
  Top 0.508: U1.41 26.54,19.23 R22.1
  Bottom 0.254: v30.23,23.22 30.23,22.61 44.96,7.87 49.4,7.87 50.8,6.48
  Bottom 1.016: PLATFORM1.A5 CON2.6 50.8,6.48
AGND  (via drill 0.6)
  Top 0.508: AGND_E.2 27.56,12.32 27.56,13.21 C10.2 | U1.43 28.96,19.38 v28.96,17.14 | U1.23 30.1,34.05 30.1,34.92 C1.2 | 13.84,47.12 14.1,46.86 20.07,46.86 22.35,44.58 22.35,41.66 | v20.32,35.31 20.32,39.62 22.35,41.66 | 22.35,41.66 v24.64,41.66
  Top 1.016: C10.2 C2.2 | C2.2 C14.2 | C2.2 v30.23,12.95 | v31.24,37.21 C1.2 | 13.84,47.12 CON4.7
  Bottom 0.508: v30.23,12.95 28.96,14.22 v28.96,17.14 28.96,18.03 22.99,24 22.99,29.84 22.61,30.23 22.61,33.4 20.7,35.31 v20.32,35.31 | v24.64,41.66 26.42,41.66 30.86,37.21 v31.24,37.21
  Bottom 1.016: PLATFORM1.GND@2 12.7,49.78 CON4.7
AREF  (via drill 0.6)
  Top 0.254: U1.42 31.11,22.67 31.11,24.26 28.96,26.42 v28.32,26.42
  Top 0.508: C10.1 27.94,16.38 27.94,19.49 U1.42
  Bottom 0.254: v28.32,26.42 28.32,26.92 27.56,27.69 27.56,29.95 20.55,36.96 17.02,36.96 15.62,38.35 15.62,42.8 11.05,47.37
  Bottom 1.016: PLATFORM1.AREF 10.16,49.78 CON4.8 11.05,47.37
D0(RXD)  (via drill 0.6)
  Top 0.254: 49.66,47.12 48.77,46.23 47.12,46.23 34.67,33.78 34.67,33.01 U1.20 33.4,31.74 v33.4,30.48
  Top 1.016: 49.66,47.12 CON3.1
  Bottom 0.254: v33.4,30.48 36.32,30.48 41.4,25.4 49.53,25.4 49.91,25.02
  Bottom 1.016: CON3.1 PLATFORM1.D0 | 49.91,25.02 UEXT.4
D1(TXD)  (via drill 0.6)
  Top 0.254: v33.38,29.21 33.02,29.21 32.38,29.84 32.38,31.86 U1.21 34.16,33.64 34.16,34.04 46.86,46.74 47.88,46.74 48.26,47.12
  Top 1.016: 48.26,47.12 CON3.2
  Bottom 0.254: v33.38,29.21 36.93,29.21 41.25,24.89 47.5,24.89 47.88,24.51
  Bottom 1.016: CON3.2 PLATFORM1.D1 | 47.88,24.51 UEXT.3
D2(SDA)  (via drill 0.6)
  Top 0.254: R12.1 46.48,22.86 49.53,22.86 | v34.21,28.35 34.31,28.45 34.31,30.84 34.16,30.99 34.16,31.37 U1.19 35.31,32.52 35.31,33.66 45.21,43.56 v45.72,43.56
  Top 1.016: UEXT.6 49.53,22.86
  Bottom 0.254: PLATFORM1.SDA 10.67,52.83 43.69,52.83 PLATFORM1.D2 | v34.21,28.35 34.44,28.57 36.91,28.57 41.1,24.38 46.23,24.38 47.75,22.86 49.53,22.86 49.91,22.48 | 45.72,46.99 v45.72,43.56
  Bottom 1.016: CON4.9 7.62,49.78 PLATFORM1.SDA | PLATFORM1.D2 CON3.3 45.72,46.99 | 49.91,22.48 UEXT.6
D3(SCL)  (via drill 0.6)
  Top 0.254: 7.75,52.45 8.13,52.83 41.15,52.83 41.53,52.45 | v35.23,27.69 35.23,29.79 34.8,30.23 34.8,30.88 U1.18 35.81,31.89 35.81,33.4 44.83,42.42 v45.34,42.42
  Top 1.016: PLATFORM1.SCL 7.75,52.45 | 41.53,52.45 PLATFORM1.D3 | UEXT.5 R11.1
  Bottom 0.254: v35.23,27.69 35.61,28.07 36.75,28.07 40.95,23.88 45.97,23.88 47.88,21.97 | 44.45,46.99 44.83,46.61 44.83,42.93 v45.34,42.42
  Bottom 1.016: CON4.10 5.08,49.78 PLATFORM1.SCL | PLATFORM1.D3 CON3.4 44.45,46.99 | 47.88,21.97 UEXT.5
D4
  Top 0.254: U1.25 28.57,33.31 28.57,42.8 32,46.23 38.61,46.23 39.5,47.12
  Top 1.016: 39.5,47.12 CON3.5
  Bottom 1.016: CON3.5 PLATFORM1.D4
D5  (via drill 0.6)
  Top 0.254: U1.31 26.78,28.32 29.84,28.32 v30.48,28.96
  Bottom 0.254: v30.48,28.96 30.48,29.49 32.64,31.65 32.64,45.47 34.16,46.99 36.83,46.99 37.21,47.37
  Bottom 1.016: PLATFORM1.D5 CON3.6 37.21,47.37
D6
  Top 0.254: U1.27 27.69,31.94 27.69,32.51 28.07,32.89 28.07,43.05 31.75,46.74 34.04,46.74 34.42,47.12
  Top 1.016: 34.42,47.12 CON3.7
  Bottom 1.016: CON3.7 PLATFORM1.D6
D7(LED1)  (via drill 0.6)
  Top 0.254: v22.61,38.73 22.61,37.59 23.24,36.96 LED1_E.2
  Top 0.508: U1.1 33.66,19.18 34.54,19.18 v34.8,19.43
  Bottom 0.254: v34.8,19.43 35.69,20.32 35.69,24.13 35.18,24.64 33.58,24.64 29.59,28.63 29.59,30.35 | 29.59,30.35 30.61,30.35 32.13,31.88 32.13,45.72 33.02,46.61 33.02,47.12 | 29.59,30.35 29.59,30.58 22.61,37.57 v22.61,38.73
  Bottom 1.016: PLATFORM1.D7 CON3.8 33.02,47.12
D8(UEXT_PWR_E)  (via drill 0.6)
  Top 0.254: 27.94,46.99 27.56,46.61 27.56,33.15 27.18,32.77 27.18,31.31 U1.28 28.65,29.84 30.79,29.84 31.62,29.01 v31.62,28.45
  Top 0.508: v41.91,26.42 42.16,26.16 FET3_E.1
  Top 1.016: 27.94,46.99 CON4.1
  Bottom 0.254: v31.62,28.45 31.62,29.9 33.1,31.37 36.09,31.37 41.05,26.42 v41.91,26.42
  Bottom 1.016: PLATFORM1.D8 27.94,49.78 CON4.1
D9(LED2)  (via drill 0.6)
  Top 0.254: U1.29 26.54,30.82 26.54,34.67 v26.67,34.8 27.05,35.18 27.05,44.83 25.4,46.48 25.4,46.99 | v23.88,37.59 24,37.47 24,33.66 23.75,33.4 LED2_E.2
  Top 1.016: 25.4,46.99 CON4.2
  Bottom 0.254: v26.67,34.8 26.04,34.8 23.88,36.96 v23.88,37.59
  Bottom 1.016: PLATFORM1.D9 25.4,49.78 CON4.2
D10
  Top 0.254: U1.30 25.78,30.45 25.78,35.13 26.54,35.89 26.54,44.58 24,47.12
  Top 1.016: 24,47.12 CON4.3
  Bottom 1.016: PLATFORM1.D10 22.86,49.78 CON4.3
D11  (via drill 0.6)
  Top 0.254: U1.12 37,26.29 35.05,26.29 31.88,29.46 31.88,31.62 v31.24,32.26
  Bottom 0.254: v31.24,32.26 31.24,33.02 20.32,43.94 20.32,47.12
  Bottom 1.016: PLATFORM1.D11 20.32,49.78 CON4.4 20.32,47.12
D12  (via drill 0.6)
  Top 0.254: U1.26 29.46,31.29 v30.35,31.29
  Bottom 0.254: v30.35,31.29 30.35,33.15 19.81,43.69 19.81,46.23 18.16,47.88
  Bottom 1.016: PLATFORM1.D12 17.78,49.78 CON4.5 18.16,47.88
D13(UEXT_#CS)  (via drill 0.6)
  Top 0.254: R13.1 46.48,20.32 48.77,20.32 49.53,19.56 49.53,17.78 | v25.65,36.45 25.27,36.07 25.27,30.1 24.89,29.72 24.89,29.07 U1.32 26.15,27.81 29.08,27.81 31.75,25.15 36.32,25.15 v36.58,25.4
  Top 1.016: UEXT.10 49.53,17.78
  Bottom 0.254: v25.65,36.45 25.65,37.08 19.3,43.43 19.3,45.97 18.29,46.99 16.51,46.99 16.13,47.37 | v36.58,25.4 38.1,23.88 38.1,23.5 39.62,21.97 44.58,21.97 46.99,19.56 46.99,18.54 47.75,17.78 48.9,17.78 50.16,16.51
  Bottom 1.016: PLATFORM1.D13 15.24,49.78 CON4.6 16.13,47.37 | 50.16,16.51 UEXT.10
D14(MISO)  (via drill 0.6)
  Top 0.254: U1.11 40.01,24.14 v40.01,22.86
  Bottom 0.254: v40.01,22.86 44.45,22.86 UEXT.7 | 46.86,40.51 46.48,40.13 46.48,36.07 52.07,30.48 52.07,18.54 51.31,17.78 50.16,17.78 48.9,19.05
  Bottom 1.016: 46.86,40.51 ICSP.1 | UEXT.7 48.9,19.05
D15(SCK)  (via drill 0.6)
  Top 0.254: U1.9 38.1,23.79 38.1,22.61 v37.85,22.35
  Bottom 0.254: v37.85,22.35 38.48,22.35 39.37,21.46 44.32,21.46 46.48,19.3 46.48,17.4 47.37,16.51 | 47.37,38.48 46.99,38.1 46.99,36.32 52.58,30.73 52.58,16.51 51.31,15.24 49.53,15.24 49.15,15.62
  Bottom 1.016: 47.37,16.51 UEXT.9 49.15,15.62 | 47.37,38.48 ICSP.3
D16(MOSI)  (via drill 0.6)
  Top 0.254: U1.10 39.12,23.9 v39.12,23.75
  Top 1.016: UEXT.8 v53.47,21.72
  Bottom 0.254: v39.12,23.75 40.39,23.75 40.77,23.37 44.7,23.37 47.75,20.32 49.53,20.32 49.91,19.94 | 49.53,38.1 49.53,34.54 53.09,30.99 53.09,22.1 v53.47,21.72
  Bottom 1.016: 49.91,19.94 UEXT.8 | 49.53,38.1 ICSP.4
D17(RXLED)  (via drill 0.6)
  Top 0.254: U1.8 36.12,24.64 31.5,24.64 28.83,27.3 27.43,27.3 v27.05,26.92 | RXLED_E.2 17.4,34.8 v18.16,35.56
  Bottom 0.254: v27.05,26.92 27.05,29.79 20.65,36.2 18.8,36.2 v18.16,35.56
D+  (via drill 0.6)
  Top 0.254: R2.2 12.57,37.85 v17.53,37.85
  Top 0.406: U1.4 34.16,22.07 34.16,23.09 33.5,23.75 32.38,23.75 v32,23.37
  Bottom 0.254: v32,23.37 32,24 28.07,27.94 28.07,30.12 20.34,37.85 v17.53,37.85
D-  (via drill 0.6)
  Top 0.254: R1.2 11.81,38.61 16.38,38.61 v16.51,38.73
  Top 0.406: U1.3 33.15,21.95 v33.15,22.73
  Bottom 0.254: v33.15,22.73 33.15,23.62 28.57,28.19 28.57,30.28 20.12,38.73 v16.51,38.73
GND  (via drill 0.6)
  Top 0.406: 51.94,33.78 51.94,33.86 50.8,35 50.8,35.08
  Top 0.508: USB.GND 9.36,35.47 C7.2 | C18.2 15.88,26.67 U2.2 | R18.1 12.95,27.56 12.32,28.19 12.32,28.83 | 12.32,28.83 10.29,28.83 C13.2 | 25.4,10.79 AGND_E.1 | 12.32,28.83 12.32,30.23 13.21,31.11 v13.59,31.11 | U1.15 38.3,30.99 40.77,30.99 v41.27,30.48 | 51.94,33.78 51.94,27.81 UEXT.2 | U1.5 39.83,17.53 45.21,17.53 | U1.35 24.53,24 C4.2 | 45.21,17.53 45.21,15.49 49.66,11.05 | 45.21,17.53 C5.1 | ICSP.6 52.32,38.35 52.32,42.55 v49.66,45.21
  Top 0.762: VR2(3.3V).1 20.22,14.5 19.68,13.97 C11.2 | 2.03,27.43 2.03,27.3 4.57,27.3 5.21,27.94 v7.87,27.94 9.14,27.94 C13.2
  Top 1.016: v0.89,44.2 TXLED.C | C13.2 C23.2 | C11.2 C12.2 19.68,11.18 | 19.68,11.18 C22.2 C20.2 C21.2 25.4,10.79 v25.4,10.03 | R18.1 13.34,26.67 14.22,25.78 C18.2 | 16.13,8.38 C16.2 | 16.13,8.38 17.53,8.38 19.68,10.54 19.68,11.18 | R10.1 v14.61,8.38 16.13,8.38 | v8.51,0.89 LED2.C LED1.C | 9.65,34.42 C7.2 | v8.51,34.42 9.65,34.42 | v13.59,31.11 14.22,31.75 C17.2 | R5.2 9.4,18.16 8.51,17.27 8.51,15.75 | 8.51,15.75 8.51,14.35 9.53,13.34 R4.1 | 3.7V-LI_BAT.2 6.37,15.75 8.51,15.75 | v0.89,27.43 2.03,27.43 RXLED.C | 9.65,34.42 C6.2 | v18.03,31.75 R6.2 | C15.2 R8.1 32.77,35.94 v33.53,35.18 | C8.1 45.97,32.13 Q1.NC_2 46.33,32.35 v47.62,33.66 | v41.27,30.48 C3.2 | v44.45,34.67 43.31,34.67 | 43.31,34.67 42.48,34.67 Q1.NC_1 42.04,34.8 v38.48,34.8 | 43.31,34.67 C9.1 | v24.77,20.57 23.62,21.72 C4.2 | CON1.5 32.26,6.86 45.47,6.86 49.66,11.05 54.74,16.13 54.74,22.73 UEXT.2 | 50.8,35.08 ICSP.6
  Bottom 1.016: CON1.4 PLATFORM1.GND PLATFORM1.GND@1 CON1.5 CON1.4 | 0.89,31.75 v0.89,27.43 0.89,17.65 3.94,14.61 | 0.89,31.75 v0.89,44.2 | 3.7V-LI_BAT.2 5.1,15.76 3.94,14.61 | 3.94,14.61 3.02,13.69 PWR.- 3.02,6.37 4.65,4.75 PWR.-- 8.51,4.75 | 8.51,4.75 10.97,4.75 v14.61,8.38 | v8.51,0.89 8.51,4.75 | 8.51,31.75 v8.51,34.42 | 0.89,31.75 8.51,31.75 | 8.51,31.75 13.59,31.75 | CON1.4 27.94,7.49 v25.4,10.03 25.78,10.03 25.78,19.56 v24.77,20.57 | 13.59,31.75 v18.03,31.75 | 13.59,31.75 v13.59,31.11 | v47.62,33.66 50.8,30.48 UEXT.2 | v44.45,34.67 46.61,34.67 v47.62,33.66 | v41.27,30.48 44.45,30.48 v47.62,33.66 | v33.53,35.18 38.1,35.18 v38.48,34.8
  other vias: 10.03,45.97 10.03,42.16 17.4,45.59 19.3,41.02 21.46,39.24 37.08,19.94 5.71,29.72 11.94,29.08 39.62,40.77 31.11,43.56 41.91,46.35 25.02,44.07 30.99,48.39 20.19,14.73
  pour Top (isolate 0.406, rank 2): -2.54,55.88 58.42,55.88 58.42,-2.54 -2.54,-2.54
  pour Bottom (isolate 0.406, rank 2): -5.08,58.42 60.96,58.42 60.96,-5.08 -5.08,-5.08
N$1
  Top 0.508: USB.D- 8.92,37.87 9.27,38.23 R1.1 9.78,38.23
N$2
  Top 0.254: R14.2 4.19,28.83 9.27,28.83 9.91,29.46 10.67,29.46 14.99,33.78 14.99,34.16 RXLED_E.1
N$3
  Top 0.508: USB.D+ 8.9,37.07 9.27,36.7 R2.1
N$4
  Top 0.508: R11_E.1 R11.2
N$5
  Top 1.016: TXLED.A R15.1
N$6  (via drill 0.6)
  Top 0.254: v47.62,31.11 48.01,31.5 48.01,32.77 48.77,33.53 R21.2
  Top 0.508: v43.18,26.42 42.93,26.16 FET3_E.2
  Bottom 0.254: v47.62,31.11 48.01,30.73 48.01,28.45 47.62,28.07 47.24,28.07 45.59,26.42 v43.18,26.42
N$8
  Top 0.508: R13_E.1 R13.2
N$9
  Top 0.254: LED1.A 6.1,3.56 8.38,3.56 8.76,3.94 10.92,3.94 11.56,4.57 R17.1
N$11  (via drill 0.6)
  Top 0.254: R8.2 35.69,36.32 37.72,38.35 v37.72,38.86
  Top 1.016: RST.P$2 44.32,40.64 v42.55,38.86
  Bottom 0.254: v37.72,38.86 v42.55,38.86
N$12
  Top 1.016: R10.2 14.61,4.7 12.19,2.29 BUT.P$1
N$13
  Top 0.508: R12_E.1 R12.2
N$15  (via drill 0.6)
  Top 0.254: LED1_E.1 21.72,33.91 19.94,33.91 v19.3,33.27 | v18.03,18.92 18.03,19.18 18.8,19.94 18.8,24.64 v18.41,25.02
  Top 0.508: R17.2 11.56,8.89 13.08,10.41 13.08,11.68 v13.34,11.94
  Bottom 0.254: v13.34,11.94 14.61,11.94 18.03,15.37 v18.03,18.92 | v19.3,33.27 19.68,32.89 19.68,26.29 v18.41,25.02
N$16
  Top 1.016: PWR.+ 9.53,11.43 D2.A
N$17
  Top 0.254: LED2.A 7.75,3.05 8.64,3.05 8.89,3.3 11.05,3.3 R16.1
N$18  (via drill 0.6)
  Top 0.254: LED2_E.1 20.95,33.4 v20.57,33.02 | v18.92,18.03 18.92,19.3 19.3,19.68 19.3,24.64 v19.68,25.02
  Top 0.508: R16.2 13.08,9.14 14.1,10.16 v14.1,10.92
  Bottom 0.254: v14.1,10.92 14.35,10.92 18.92,15.49 v18.92,18.03 | v20.57,33.02 20.19,32.64 20.19,25.53 v19.68,25.02
N$19
  Top 0.254: FET3.1 46.29,27.11 47.24,28.07 48.26,28.07 C19.2
  Top 1.016: C19.2 R20.2 R21.1
N$20
  Top 1.016: FET3.2 44.2,27.2 R19.2
N$21
  Top 1.016: R5.1 PWR_LED.C
N$22
  Top 0.508: U2.5 14,30 R18.2
N$23
  Top 1.016: RXLED.A R14.1
N$118
  Top 1.016: USB.GND3 2.5,32.64 3.05,32.64 | USB.GND1 2.5,41.66 3.05,41.66 3.05,41.53 | 3.05,32.64 3.05,41.53 | USB.GND2 6.75,41.53 3.05,41.53 | 3.05,32.64 6.75,32.64 USB.GND4 6.75,31.88 10.29,31.88 11.43,33.02 C6.1
RESET  (via drill 0.6)
  Top 0.508: v39.52,29.26 38.84,29.26 U1.13 36.76,27.18 v36.32,27.18 | v41.66,37.85 47.24,37.85 47.5,37.59 | v35.94,18.92 35.94,18.54 34.29,16.89 34.29,12.06 30.23,8 21.46,8 20.32,6.86 20.32,6.48
  Top 1.016: D1.A 36.19,41.27 35.56,40.64 | 35.56,40.64 34.54,39.62 R7.2 C15.1 v35.94,37.85 | 35.56,40.64 RST.P$1 | 47.5,37.59 ICSP.5 | CON1.1 20.32,6.48
  Bottom 0.254: v36.32,27.18 35.56,26.42 35.56,25.02 36.2,24.38 36.2,19.18 v35.94,18.92
  Bottom 0.508: 39.52,37.85 v35.94,37.85 | 39.52,37.85 v41.66,37.85 | v39.52,29.26 39.52,37.85
  Bottom 1.016: PLATFORM1.RST CON1.1
TXLED  (via drill 0.6)
  Top 0.254: R15.2 3.94,44.32 v21.21,44.32
  Top 0.508: U1.22 32.02,34.67 v31.24,34.67
  Bottom 0.254: v31.24,34.67 30.35,34.67 21.21,43.81 v21.21,44.32
UCAP
  Top 0.508: U1.6 39.95,18.54 C5.2
V+
  Top 0.508: R13_E.2 R11_E.2 R12_E.2 42.16,23.75 42.42,24 43.43,24 44.24,24.81 FET3.3 45.8,25.27 46.86,25.27 47.12,25.53
  Top 1.016: 47.12,25.53 UEXT.1
VBAT  (via drill 0.6)
  Top 0.508: C18.1 16.82,25.84 U2.3 16.92,27.3 19.52,27.3 FET2.3
  Top 0.762: v16.76,24.64 C18.1
  Bottom 0.254: 4.83,25.02 6.6,25.02
  Bottom 0.762: 3.7V-LI_BAT.1 5.86,17.76 4.06,19.56 4.06,24.51 4.57,25.02 4.83,25.02 | 6.6,25.02 6.86,25.02 8.26,23.62 10.82,23.62 11.84,24.64 v16.76,24.64
VBUS
  Top 0.508: USB.VBUS 7.94,38.67 9.78,40.51 L1.1
VCC  (via drill 0.6)
  Top 0.508: U1.14 38.7,30.25 39.98,30.25 v41.27,28.96 | D1.C v33.66,41.4 | U1.34 24.41,25.02 22.86,25.02 C4.1
  Top 0.762: R9.1 19.18,7.11 20.95,8.89 24.13,8.89 | 24.13,8.89 v24.13,9.65 | 24.13,8.89 27.69,8.89 v28.19,9.4 28.85,10.06 L2.1 | v39.5,20.57 41.27,22.35 41.27,25.4 40.77,25.91 40.77,28.45 v41.27,28.96
  Top 1.016: R22.2 R23.2 24.51,16.76 v24.51,15.88 | D1.C 32.39,39.87 R7.1 | R20.1 C19.1 48.9,30.1 47.75,28.96 v47.12,28.96 46.23,28.96 R19.1 | C3.1 42.42,28.96 v41.27,28.96 | v20.7,23.5 21.21,24 C4.1 | v35.31,12.45 35.31,16.38 v37.34,18.41
  Bottom 0.508: 49.91,42.8 49.4,43.31 47.12,43.31 46.74,42.93 46.74,42.29 45.85,41.4 | v41.27,28.96 40.26,29.97 40.26,32 45.85,37.59 45.85,41.4 | 45.85,41.4 44.83,41.4 44.32,41.91 34.16,41.91 v33.66,41.4
  Bottom 1.016: v41.27,28.96 v47.12,28.96 | 49.91,42.8 ICSP.2 | 3.3V/5V.2 6.35,23.75 7.62,22.48 11.3,22.48 12.19,23.37 20.7,23.37 | 20.7,23.37 v20.7,23.5 | 20.7,23.37 20.7,21.72 24.13,18.29 24.13,15.88 | v24.13,9.65 24.13,15.88 | 24.13,15.88 v24.51,15.88 | v28.19,9.4 32.26,9.4 v35.31,12.45 | v37.34,18.41 v39.5,20.57
VDD  (via drill 0.6)
  Top 0.508: U1.44 29.97,19.26 29.97,17.65 v30.23,17.4 | U1.24 29.34,33.68 29.34,35.94 C1.1 | v24,29.72 24.64,30.35 24.64,36.83 25.91,38.1 25.91,40.39 v25.65,40.64
  Top 1.016: L2.2 32.13,11.81 33.27,12.95 33.27,15.49 32.89,15.88 C14.1 C2.1 v30.23,17.4 | v29.46,37.21 C1.1
  Bottom 0.508: v30.23,17.4 30.23,17.91 23.75,24.38 23.75,29.46 v24,29.72 | v25.65,40.64 26.29,40.64 29.46,37.47 v29.46,37.21
VR1_ADJ
  Top 1.016: 13.56,13.34 R3.1 | 13.56,13.34 VR1(5.0V).1 | R4.2 13.56,13.34
XTAL1
  Top 0.508: U1.17 38.71,33.66 44.9,33.66 Q1.1
  Top 1.016: Q1.1 45.09,36.07 C9.2
XTAL2
  Top 0.508: U1.16 38.95,32.77 41.78,32.77 Q1.2
  Top 1.016: Q1.2 42.96,32.35 44.2,31.11 C8.2

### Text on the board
tNames: WWW.OLIMEX.COM/DEV | Rev.A | OLIMEXINO-32U4
bNames: MADE IN BULGARIA BY:
